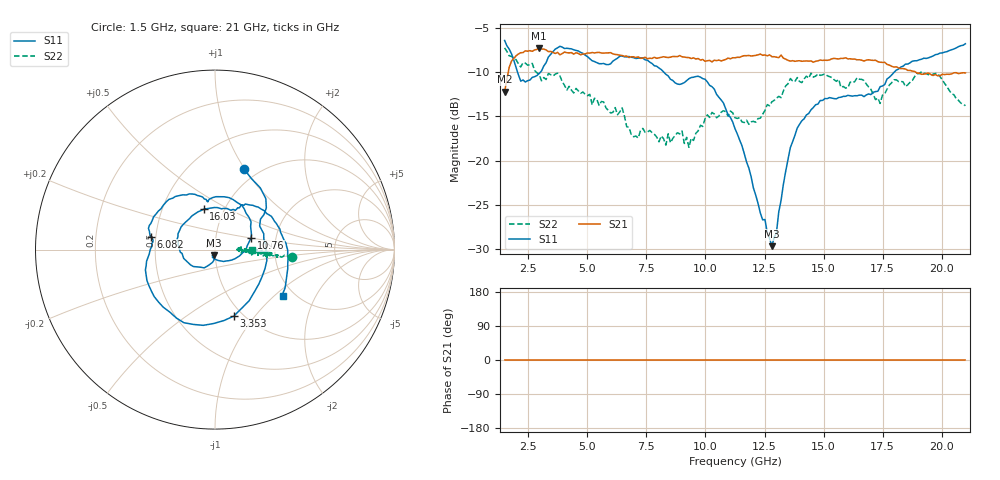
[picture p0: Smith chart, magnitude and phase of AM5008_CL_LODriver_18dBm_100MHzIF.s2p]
!Keysight Technologies,N5245B,MY58422270,A.16.20.02
!Mixer S2P File: Scalar Mixer Measurement
!Calibration State: On
!Parameters: Stimulus Freq, S11, SC21, SC12, S22
# Hz  S  DB  R  50.0
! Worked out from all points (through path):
!   201 points, 1.5 GHz to 21 GHz, reference 50 ohm
!   highest |S21| = -7.31 dB at 2.962 GHz (marker M1); lowest = -12.2 dB at 1.5 GHz (marker M2)
!   lowest |S11| = -29.7 dB at 12.81 GHz (marker M3), VSWR 1.07, Z = 49.1 - j3.14 ohm
!   |S11| at or under -10 dB: 2.049 GHz to 3.017 GHz (968.2 MHz wide, 38.2 % of centre); 8.238 GHz to 17.99 GHz (9.752 GHz wide, 74.4 % of centre)
!   |S22| runs from -18.5 to -7.3 dB; largest |S21 - S12| = 0.43
!   S11 on the Smith chart (normalised r, x): 1.5 GHz: 0.85, +0.99; 3.353 GHz: 0.91, -0.79; 6.082 GHz: 0.47, +0.08; 10.76 GHz: 1.49, +0.20; 16.03 GHz: 0.80, +0.38; 21 GHz: 1.74, -1.14
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1.5e9  -6.42 70.3  -12.22 0.0  -200.00 90.0  -7.26 -5.2
1.7925e9  -7.93 45.1  -8.75 0.0  -200.00 90.0  -8.22 -4.6
2.1825e9  -11.02 27.8  -7.81 0.0  -200.00 90.0  -9.42 -5.1
2.9625e9  -10.16 -38.0  -7.31 0.0  -200.00 90.0  -10.24 -5.0
3.3525e9  -8.29 -74.3  -7.68 0.0  -200.00 90.0  -10.16 -4.3
4.1325e9  -7.30 -131.9  -7.81 0.0  -200.00 90.0  -12.03 -3.0
4.815e9  -7.88 -163.8  -7.95 0.0  -200.00 90.0  -12.25 -6.2
6.0825e9  -8.76 168.5  -7.94 0.0  -200.00 90.0  -14.55 -1.1
8.0325e9  -9.53 111.9  -8.38 0.0  -200.00 90.0  -17.86 -1.8
9.3e9  -10.74 92.3  -8.36 0.0  -200.00 90.0  -18.49 3.2
9.69e9  -10.46 74.9  -8.46 0.0  -200.00 90.0  -16.65 -1.0
1.07625e10  -13.49 18.1  -8.64 0.0  -200.00 90.0  -14.36 -2.4
1.125e10  -16.39 -8.6  -8.38 0.0  -200.00 90.0  -15.15 -4.1
1.281e10  -29.65 -104.1  -8.26 0.0  -200.00 90.0  -13.35 -5.2
1.359e10  -18.54 -120.7  -8.75 0.0  -200.00 90.0  -10.72 -6.0
1.4565e10  -14.00 177.5  -8.88 0.0  -200.00 90.0  -10.57 -6.1
1.60275e10  -12.62 105.8  -8.50 0.0  -200.00 90.0  -11.77 -3.2
1.66125e10  -12.60 86.5  -8.65 0.0  -200.00 90.0  -10.82 -5.3
1.73925e10  -11.64 61.6  -8.88 0.0  -200.00 90.0  -13.53 -4.0
1.77825e10  -10.58 56.7  -9.20 0.0  -200.00 90.0  -11.45 -4.6
1.983e10  -7.98 2.7  -10.42 0.0  -200.00 90.0  -10.15 -4.3
2.1e10  -6.79 -34.4  -10.09 0.0  -200.00 90.0  -13.79 -0.5
